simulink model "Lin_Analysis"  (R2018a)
settings: Solver=ode4  StartTime=0.0  StopTime=40000  FixedStep=Ts  MaxStep=0.5  RelTol=1e-3  EnableMultiTasking=on
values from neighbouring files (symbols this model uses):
  Int_IC = [qti', 0 0, h0i(1:3)', 0 0, wr0, Vec0'*M0, Pec0']    [run.m]
  Kq1 = I22*ww^2 - 3*wo2*(I11-I33)    [run.m]
  Kq2 = 2*I22*zet*ww    [run.m]
  Kqi = 0.0005    [run.m]
  Kr1 = (0.1*I11*I33*zet^2/Hy0) - sqrt( ((0.01^zet^4*I11^2*I33^2)/Hy0^2)+(4*I11*I33*zet^2) )    [run.m]
  Kr2 = 0.05*Kr1    [run.m]
  Kr3 = 0.04*zet*(Kr2-Hy0) * sqrt(abs(Hy0/(I11*I33)))    [run.m]
  nt = 7    [run.m]    (also in runf.m)
  r2d = 180/pi    (= 57.2957795131)    [pl.m]    (also in pl2.m; run.m; plf.m; runf.m)
  Ts = 0.001    [run.m]    (also in runf.m = 0.0005)
undefined symbols (not defined in the file or in its folder): Aflx, Bflx, Cflx, den, Dflx, DiscIntNeverNeededParam, num, RW_Steering, Vehi_3B3W
libraries: simulink x3

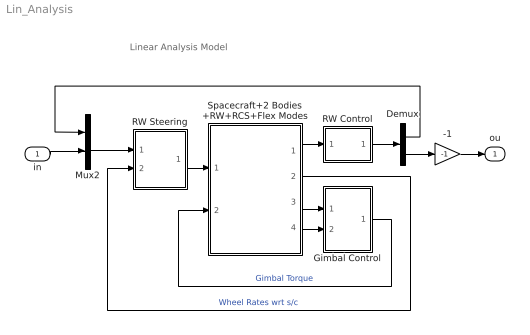
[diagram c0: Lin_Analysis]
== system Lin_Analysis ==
  note: Linear Analysis Model
  in : Inport
  -1 : Gain  Gain=-1
  Demux : Demux  Outputs=2
  Gimbal Control : Subsystem
  Mux2 : Mux  Inputs=2
  RW Control : Subsystem
  RW Steering : Subsystem
  Spacecraft+2 Bodies +RW+RCS+Flex Modes : Subsystem
  ou : Outport
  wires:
  Spacecraft+2 Bodies +RW+RCS+Flex Modes/1(atti) -> RW Control/1(atti)
  Spacecraft+2 Bodies +RW+RCS+Flex Modes/2(Wrw) -> RW Steering/2(wr(1))  "Wheel Rates wrt s/c"
  Spacecraft+2 Bodies +RW+RCS+Flex Modes/4(Gmb-dot) -> Gimbal Control/2(Grat)
  RW Steering/1(Twi) -> Spacecraft+2 Bodies +RW+RCS+Flex Modes/1(Trw)
  -1/1 -> ou/1
  Gimbal Control/1(GTrq) -> Spacecraft+2 Bodies +RW+RCS+Flex Modes/2(Tgimb)  "Gimbal Torque"
  Spacecraft+2 Bodies +RW+RCS+Flex Modes/3(gimb) -> Gimbal Control/1(Gimb)
  RW Control/1(Tc) -> Demux/1
  Mux2/1 -> RW Steering/1(Trwc)
  Demux/2 -> -1/1
  in/1 -> Mux2/2
  Demux/1 -> Mux2/1

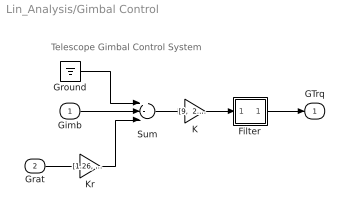
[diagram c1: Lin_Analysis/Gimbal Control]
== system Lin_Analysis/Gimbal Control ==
  note: Telescope Gimbal Control System
  Gimb : Inport
  Grat : Inport  Port=2
  Filter : Subsystem
  Ground : Ground
  K : Gain  Gain="[9,  2.85]"
  Kr : Gain  Gain="[1.26,  1.14]"
  Sum : Sum  Inputs=+--
  GTrq : Outport
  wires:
  Filter/1(O) -> GTrq/1
  Sum/1 -> K/1
  Gimb/1 -> Sum/2
  Grat/1 -> Kr/1
  Kr/1 -> Sum/3
  Ground/1 -> Sum/1
  K/1 -> Filter/1(I)

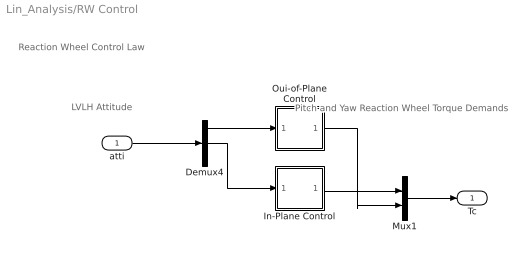
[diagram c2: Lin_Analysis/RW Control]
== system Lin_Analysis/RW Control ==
  note: Pitch and Yaw Reaction Wheel Torque Demands
  note: LVLH Attitude
  note: Reaction Wheel Control Law
  atti : Inport
  Demux4 : Demux  Outputs=3
  In-Plane Control : Subsystem
  Mux1 : Mux  Inputs=2
  Oui-of-Plane Control : Subsystem
  Tc : Outport
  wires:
  Demux4/1 -> Oui-of-Plane Control/1(phi)
  In-Plane Control/1(Tcy) -> Mux1/1
  Demux4/2 -> In-Plane Control/1(the)
  Oui-of-Plane Control/1(Tcz) -> Mux1/2
  atti/1 -> Demux4/1
  Mux1/1 -> Tc/1

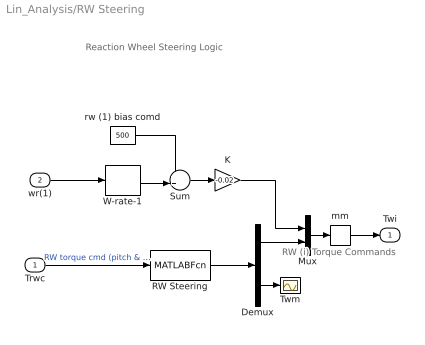
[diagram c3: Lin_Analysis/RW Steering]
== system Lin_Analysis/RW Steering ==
  note: Reaction Wheel Steering Logic
  note: RW (i) Torque Commands
  Trwc : Inport
  wr(1) : Inport  Port=2
  Demux : Demux  Outputs=[2, 1]
  K : Gain  Gain=-0.02
  Mux : Mux  Inputs=[1,2]
  RW Steering : MATLABFcn  MATLABFcn=RW_Steering( u(1:2) )  OutputDimensions=3
  Sum : Sum  Inputs=++|
  Twm : Scope
  W-rate-1 : Selector  InputPortWidth=3  IndexOptions=Index vector (dialog)  Indices=[1]  OutputSizes=1
  mm : Memory
  rw (1) bias comd : Constant  Value=500
  Twi : Outport
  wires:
  K/1 -> Mux/1
  W-rate-1/1 -> Sum/2
  rw (1) bias comd/1 -> Sum/1
  Sum/1 -> K/1
  wr(1)/1 -> W-rate-1/1
  Mux/1 -> mm/1
  Trwc/1 -> RW Steering/1  "RW torque cmd (pitch & yaw)"
  RW Steering/1 -> Demux/1
  Demux/1 -> Mux/2
  Demux/2 -> Twm/1
  mm/1 -> Twi/1

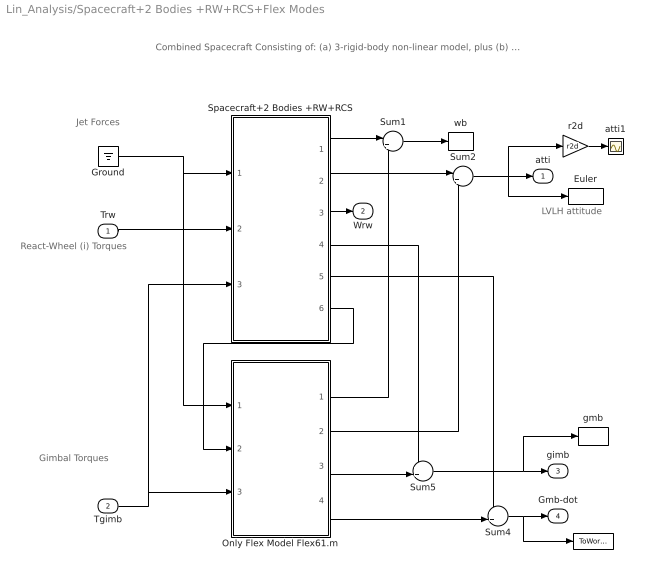
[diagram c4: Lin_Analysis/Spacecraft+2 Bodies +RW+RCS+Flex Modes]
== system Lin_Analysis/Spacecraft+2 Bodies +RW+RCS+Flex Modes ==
  note: React-Wheel (i) Torques
  note: Jet Forces
  note: Gimbal Torques
  note: Combined Spacecraft Consisting of: (a) 3-rigid-body non-linear model, plus (b) a 61 flex modes state-space model
  note: LVLH attitude
  Trw : Inport
  Tgimb : Inport  Port=2
  "   " : ToWorkspace  VariableName=Gimdot  SampleTime=-1
  Euler : ToWorkspace  VariableName=Euler  SampleTime=-1
  Ground : Ground
  Only Flex Model Flex61.m : Subsystem
  Spacecraft+2 Bodies +RW+RCS : Subsystem
  Sum1 : Sum  Inputs=|++
  Sum2 : Sum  Inputs=|++
  Sum4 : Sum  Inputs=++|
  Sum5 : Sum  Inputs=++|
  atti1 : Scope
  gmb : ToWorkspace  VariableName=Gimb  SampleTime=-1
  r2d : Gain  Gain=r2d
  wb : ToWorkspace  VariableName=wb  SampleTime=-1
  atti : Outport
  Wrw : Outport  Port=2
  gimb : Outport  Port=3
  Gmb-dot : Outport  Port=4
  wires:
  Spacecraft+2 Bodies +RW+RCS/6(Twb) -> Only Flex Model Flex61.m/2(Trwb)
  Only Flex Model Flex61.m/1(wb) -> Sum1/2
  Only Flex Model Flex61.m/4(Gmb-dot) -> Sum4/2
  Only Flex Model Flex61.m/3(gimb) -> Sum5/2
  Only Flex Model Flex61.m/2(atti) -> Sum2/2
  r2d/1 -> atti1/1
  Sum4/1 -> "   "/1, Gmb-dot/1
  Sum5/1 -> gmb/1, gimb/1
  Sum2/1 -> r2d/1, Euler/1, atti/1
  Sum1/1 -> wb/1
  Spacecraft+2 Bodies +RW+RCS/3(Wrw) -> Wrw/1
  Spacecraft+2 Bodies +RW+RCS/5(Gmb-dot) -> Sum4/1
  Spacecraft+2 Bodies +RW+RCS/4(gimb) -> Sum5/1
  Spacecraft+2 Bodies +RW+RCS/2(att) -> Sum2/1
  Spacecraft+2 Bodies +RW+RCS/1(W_b) -> Sum1/1
  Tgimb/1 -> Only Flex Model Flex61.m/3(Tgimb), Spacecraft+2 Bodies +RW+RCS/3(Tgimb)
  Trw/1 -> Spacecraft+2 Bodies +RW+RCS/2(Trw)
  Ground/1 -> Only Flex Model Flex61.m/1(Fjets), Spacecraft+2 Bodies +RW+RCS/1(Frcs)

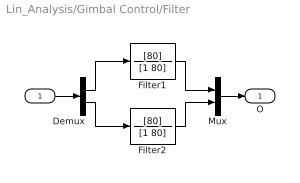
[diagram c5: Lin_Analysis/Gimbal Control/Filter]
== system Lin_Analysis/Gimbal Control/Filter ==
  I : Inport
  Demux : Demux  Outputs=2
  Filter1 : TransferFcn  Numerator=[80]  Denominator=[1 80]
  Filter2 : TransferFcn  Numerator=[80]  Denominator=[1 80]
  Mux : Mux  Inputs=2
  O : Outport
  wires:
  Filter1/1 -> Mux/1
  Filter2/1 -> Mux/2
  Demux/1 -> Filter1/1
  Demux/2 -> Filter2/1
  I/1 -> Demux/1
  Mux/1 -> O/1

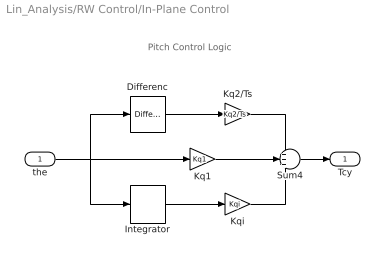
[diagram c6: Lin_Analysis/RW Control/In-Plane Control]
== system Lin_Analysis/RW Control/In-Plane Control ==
  note: Pitch Control Logic
  the : Inport
  Differenc : simulink/Discrete/Difference  ICPrevInput=0.0  InputProcessing=Inherited  OutMin=[]  OutMax=[]  OutDataType=sfix(16)  OutScaling=2^-10  DoSatur=off
  Integrator : DiscreteIntegrator  SampleTime=Ts  ICPrevOutput=DiscIntNeverNeededParam  ICPrevScaledInput=DiscIntNeverNeededParam
  Kq1 : Gain  Gain=Kq1
  Kq2/Ts : Gain  Gain=Kq2/Ts
  Kqi : Gain  Gain=Kqi
  Sum4 : Sum  Inputs=+++
  Tcy : Outport
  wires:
  Kq1/1 -> Sum4/2
  Sum4/1 -> Tcy/1
  Kq2/Ts/1 -> Sum4/1
  the/1 -> Kq1/1, Integrator/1, Differenc/1
  Kqi/1 -> Sum4/3
  Integrator/1 -> Kqi/1
  Differenc/1 -> Kq2/Ts/1

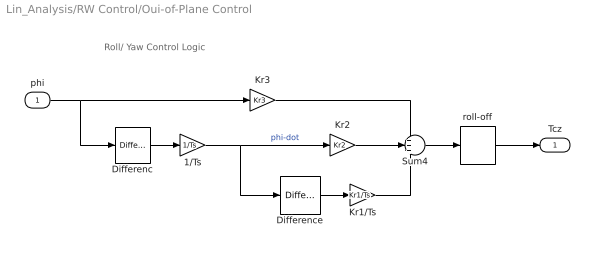
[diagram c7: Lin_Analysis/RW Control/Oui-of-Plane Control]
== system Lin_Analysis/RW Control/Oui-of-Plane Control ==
  note: Roll/ Yaw Control Logic
  phi : Inport
  1/Ts : Gain  Gain=1/Ts
  Differenc : simulink/Discrete/Difference  ICPrevInput=0.0  InputProcessing=Inherited  OutMin=[]  OutMax=[]  OutDataType=sfix(16)  OutScaling=2^-10  DoSatur=off
  Difference : simulink/Discrete/Difference  ICPrevInput=0.0  InputProcessing=Inherited  OutMin=[]  OutMax=[]  OutDataType=sfix(16)  OutScaling=2^-10  DoSatur=off
  Kr1/Ts : Gain  Gain=Kr1/Ts
  Kr2 : Gain  Gain=Kr2
  Kr3 : Gain  Gain=Kr3
  Sum4 : Sum  Inputs=+++
  roll-off : DiscreteTransferFcn  Numerator=[num]  Denominator=[den]  SampleTime=Ts
  Tcz : Outport
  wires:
  roll-off/1 -> Tcz/1
  Kr3/1 -> Sum4/1
  Kr2/1 -> Sum4/2
  Kr1/Ts/1 -> Sum4/3
  phi/1 -> Kr3/1, Differenc/1
  Sum4/1 -> roll-off/1
  Difference/1 -> Kr1/Ts/1
  Differenc/1 -> 1/Ts/1
  1/Ts/1 -> Kr2/1, Difference/1  "phi-dot"

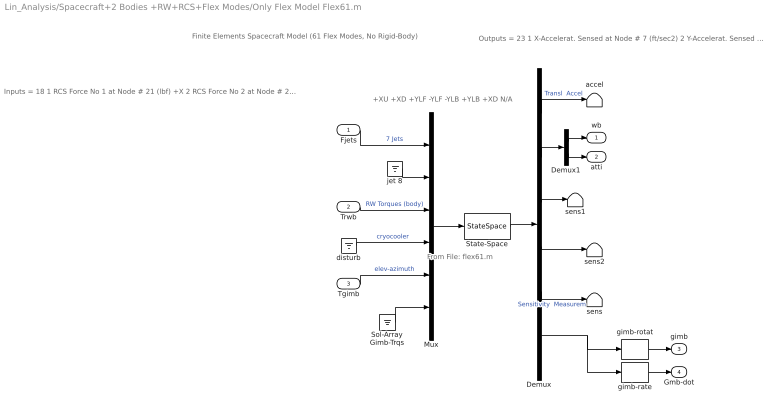
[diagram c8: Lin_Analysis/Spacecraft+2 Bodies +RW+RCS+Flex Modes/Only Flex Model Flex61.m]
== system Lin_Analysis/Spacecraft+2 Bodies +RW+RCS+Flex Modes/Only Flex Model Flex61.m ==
  note: Finite Elements Spacecraft Model (61 Flex Modes, No Rigid-Body)
  note: Inputs = 18 1 RCS Force No 1 at Node # 21 (lbf) +X 2 RCS Force No 2 at Node # 22 (lbf) +X 3 RCS Force No 3 at Node # 23 (lbf) +Y 4 RCS Force No 4 at Node # 24 (lbf) -Y 5 RCS Force No 5 at Node # 25 (lbf) -Y 6 RCS Force No 6 at Node # 26 (lbf) +Y 7 RCS Force No 7 at Node # 27 (lbf) +X 8 RCS Force No 8 at Node # 28 (lbf) +X 9 RW Torque No 1 at Node # 17 (ft-lb) roll 10 RW Torque No 2 at Node # 18 (ft-lb) ptch 11 RW Torque No 3 at Node # 19 (ft-lb) yaw 12 Dist Trque No 4 at Node # 8 (ft-lb) roll 13 Dist Trque No 5 at Node # 8 (ft-lb) ptch 14 Dist Trque No 6 at Node # 8 (ft-lb) yaw 15 Elevation Trqu at Gimbal No 1 (ft-lb) 16 Azimuth Torque at Gimbal No 2 (ft-lb) 17 Rght SA Torque at Gimbal No 3 (ft-lb) 18 Left SA Torque at Gimbal No 4 (ft-lb)
  note: Outputs = 23 1 X-Accelerat. Sensed at Node # 7 (ft/sec2) 2 Y-Accelerat. Sensed at Node # 7 (ft/sec2) 3 X-Rot. Rate Sensed at Node # 6 (radian) 4 Y-Rot. Rate Sensed at Node # 6 (radian) 5 Z-Rot. Rate Sensed at Node # 6 (radian) 6 X-Rotation Sensed at Node # 6 (radian) 7 Y-Rotation Sensed at Node # 6 (radian) 8 Z-Rotation Sensed at Node # 6 (radian) 9 Y-Rotation Mirror at Node # 9 (radian) 10 Z-Rotation Mirror at Node # 9 (radian) 11 Y-Rotation Instrum-2 Node # 10 (radian) 12 Z-Rotation Instrum-2 Node # 10 (radian) 13 X-Rotation Instrum-3 Node # 11 (radian) 14 Y-Rotation Instrum-4 Node # 12 (radian) 15 Z-Rotation Instrum-5 Node # 13 (radian) 16 Rotation Angle at Elevati Gimbal No 1 17 Rotation Rate at Elevati Gimbal No 1 18 Rotation Angle at Azimuth Gimbal No 2 19 Rotation Rate at Azimuth Gimbal No 2 20 Rotation Angle at Rght SA Gimbal No 3 21 Rotation Rate at Rght SA Gimbal No 3 22 Rotation Angle at Left SA Gimbal No 4 23 Rotation Rate at Left SA Gimbal No 4
  note: +XU +XD +YLF -YLF -YLB +YLB +XD N/A
  note: From File: flex61.m
  Fjets : Inport
  Trwb : Inport  Port=2
  Tgimb : Inport  Port=3
  Demux : Demux  Outputs="[2, 6, 2,2,3,  8]"
  Demux1 : Demux  Outputs=[3, 3]
  Mux : Mux  Inputs=[7,1,3,3,2,2]
  Sol-Array Gimb-Trqs : Ground
  State-Space : StateSpace  A=Aflx  B=Bflx  C=Cflx  D=Dflx  InitialCondition=0
  accel : Terminator
  disturb : Ground
  gimb-rate : Selector  InputPortWidth=8  IndexOptions=Index vector (dialog)  Indices=[2, 4]  OutputSizes=1
  gimb-rotat : Selector  InputPortWidth=8  IndexOptions=Index vector (dialog)  Indices=[1 3]  OutputSizes=1
  jet 8 : Ground
  sens : Terminator
  sens1 : Terminator
  sens2 : Terminator
  wb : Outport
  atti : Outport  Port=2
  gimb : Outport  Port=3
  Gmb-dot : Outport  Port=4
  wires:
  gimb-rotat/1 -> gimb/1
  gimb-rate/1 -> Gmb-dot/1
  Demux/4 -> sens2/1
  Demux/3 -> sens1/1
  Demux/6 -> gimb-rotat/1, gimb-rate/1
  Tgimb/1 -> Mux/5  "elev-azimuth"
  Demux/1 -> accel/1  "Transl  Accel"
  State-Space/1 -> Demux/1
  Demux/2 -> Demux1/1
  Demux1/1 -> wb/1
  Mux/1 -> State-Space/1
  Fjets/1 -> Mux/1  "7 Jets"
  jet 8/1 -> Mux/2
  Trwb/1 -> Mux/3  "RW Torques (body)"
  disturb/1 -> Mux/4  "cryocooler"
  Sol-Array Gimb-Trqs/1 -> Mux/6
  Demux/5 -> sens/1  "Sensitivity  Measurem"
  Demux1/2 -> atti/1

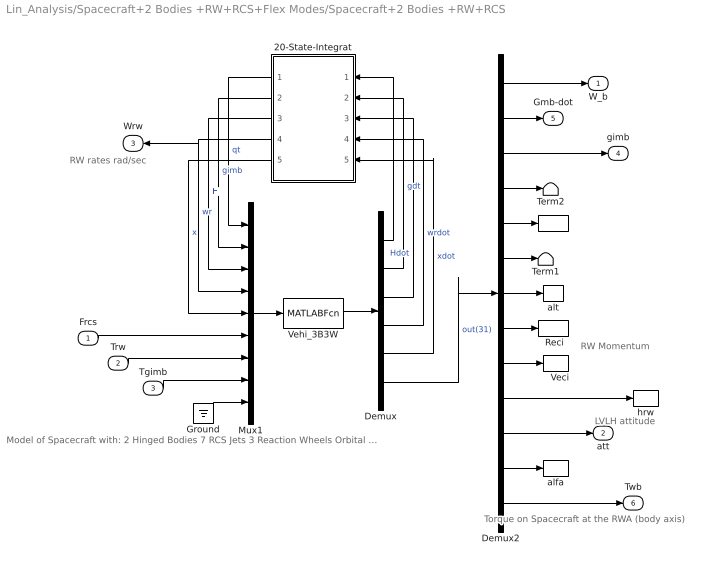
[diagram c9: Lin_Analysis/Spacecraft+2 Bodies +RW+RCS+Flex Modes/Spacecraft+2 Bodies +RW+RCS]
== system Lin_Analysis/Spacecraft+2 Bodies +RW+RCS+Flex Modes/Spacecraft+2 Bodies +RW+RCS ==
  note: RW rates rad/sec
  note: Torque on Spacecraft at the RWA (body axis)
  note: LVLH attitude
  note: Model of Spacecraft with: 2 Hinged Bodies 7 RCS Jets 3 Reaction Wheels Orbital Dynamics
  note: RW Momentum
  Frcs : Inport
  Trw : Inport  Port=2
  Tgimb : Inport  Port=3
  "    " : ToWorkspace  VariableName=hsys  SampleTime=-1
  "   Veci" : ToWorkspace  VariableName=Veci  SampleTime=-1
  "  Reci " : ToWorkspace  VariableName=Reci  SampleTime=-1
  20-State-Integrat : Subsystem
  Demux : Demux  Outputs="[4,2,5,3,6,  31]"
  Demux2 : Demux  Outputs=[3,2,2,1, 3,2, 1,3,3,3,3, 2,3]
  Ground : Ground
  Mux1 : Mux  Inputs="[4,2,5,3,6,  nt,3,2,3]"
  Term1 : Terminator
  Term2 : Terminator
  Vehi_3B3W : MATLABFcn  MATLABFcn=Vehi_3B3W( u(1:20), u(21:20+nt), u(21+nt:23+nt), u(24+nt:25+nt), u(26+nt:28+nt) )  OutputDimensions=51
  alfa : ToWorkspace  VariableName=alfa  SampleTime=-1
  alt : ToWorkspace  VariableName=alt  SampleTime=-1
  hrw : ToWorkspace  VariableName=hrw  SampleTime=-1
  W_b : Outport
  att : Outport  Port=2
  Wrw : Outport  Port=3
  gimb : Outport  Port=4
  Gmb-dot : Outport  Port=5
  Twb : Outport  Port=6
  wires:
  Frcs/1 -> Mux1/6
  Demux2/13 -> Twb/1
  Mux1/1 -> Vehi_3B3W/1
  Trw/1 -> Mux1/7
  Tgimb/1 -> Mux1/8
  Demux2/3 -> gimb/1
  Demux2/2 -> Gmb-dot/1
  Demux2/4 -> Term2/1
  Demux2/1 -> W_b/1
  Demux2/6 -> Term1/1
  Demux2/5 -> "    "/1
  Demux2/7 -> alt/1
  Demux2/8 -> "  Reci "/1
  Demux2/10 -> hrw/1
  Demux2/11 -> att/1
  Demux2/12 -> alfa/1
  Demux/5 -> 20-State-Integrat/5(xdot)  "xdot"
  Demux/4 -> 20-State-Integrat/4(wrdor)  "wrdot"
  Demux/3 -> 20-State-Integrat/3(Hdot)  "Hdot"
  Demux/2 -> 20-State-Integrat/2(gmbdot)  "gdt"
  Demux/1 -> 20-State-Integrat/1(qdot)
  Demux/6 -> Demux2/1  "out(31)"
  20-State-Integrat/5(x) -> Mux1/5  "x"
  20-State-Integrat/4(wr) -> Mux1/4, Wrw/1  "wr"
  20-State-Integrat/3(H) -> Mux1/3  "H"
  20-State-Integrat/2(gimb) -> Mux1/2  "gimb"
  20-State-Integrat/1(qt) -> Mux1/1  "qt"
  Vehi_3B3W/1 -> Demux/1
  Demux2/9 -> "   Veci"/1
  Ground/1 -> Mux1/9

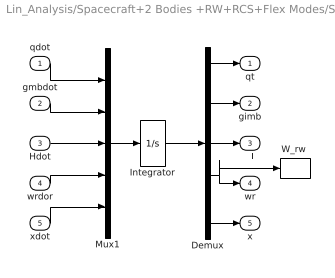
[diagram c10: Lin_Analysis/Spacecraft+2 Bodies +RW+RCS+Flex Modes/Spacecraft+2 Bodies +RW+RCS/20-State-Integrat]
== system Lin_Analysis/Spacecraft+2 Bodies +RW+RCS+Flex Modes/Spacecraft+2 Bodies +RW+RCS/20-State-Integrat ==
  qdot : Inport
  gmbdot : Inport  Port=2
  Hdot : Inport  Port=3
  wrdor : Inport  Port=4
  xdot : Inport  Port=5
  Demux : Demux  Outputs=[4,2,5,3,6]
  Integrator : Integrator  InitialCondition=Int_IC
  Mux1 : Mux  Inputs=[4,2,5,3,6]
  "W_rw " : ToWorkspace  VariableName=W_rw  SampleTime=-1
  qt : Outport
  gimb : Outport  Port=2
  H : Outport  Port=3
  wr : Outport  Port=4
  x : Outport  Port=5
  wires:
  Mux1/1 -> Integrator/1
  Integrator/1 -> Demux/1
  qdot/1 -> Mux1/1
  gmbdot/1 -> Mux1/2
  Hdot/1 -> Mux1/3
  wrdor/1 -> Mux1/4
  xdot/1 -> Mux1/5
  Demux/1 -> qt/1
  Demux/2 -> gimb/1
  Demux/3 -> H/1
  Demux/4 -> "W_rw "/1, wr/1
  Demux/5 -> x/1
